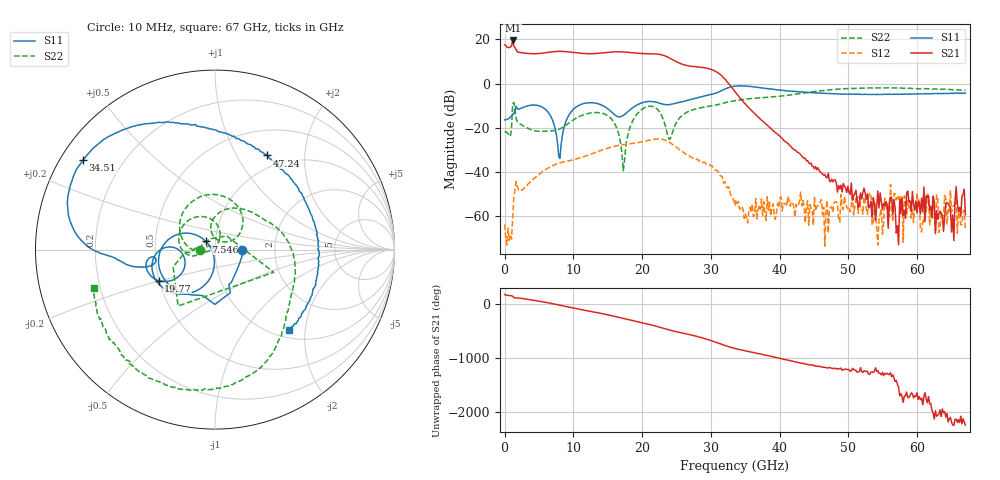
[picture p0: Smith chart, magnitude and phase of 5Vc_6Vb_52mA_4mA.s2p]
! MARKI MICROWAVE INC.
! Date:  05/05/2020
! Model Number:  APM-7099CH
! Description:  2-port Small Signal S-parameter data for APM-7099CH
! Frequency Range:  10 MHz to 67 GHz
! Port Configuration:  PORT 1: Input
!  PORT 2: Output
! Bias Condition: Vc = +5V, Vb = +6V
! APM-7099CH s2p files are only valid for small signal conditions (below -5 dBm input power)
!S2P File: Measurements: Mag<S11> Ang<S11>, Mag<S21> Ang<S21>, Mag<S12> Ang<S12>, Mag<S22> Ang<S22>!row 1
# Hz S  dB  R 50
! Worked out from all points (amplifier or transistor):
!   401 points, 10 MHz to 67 GHz, reference 50 ohm
!   highest |S21| = 19.6 dB at 1.182 GHz (marker M1)
!   |S21| within 3 dB of that: start of sweep to 376.6 MHz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
!   unconditionally stable (mu >= 1): start of sweep to end of sweep
!   at 11.06 GHz: K = 4.23, MAG = 14.4 dB, |S12| = -33.5 dB
!   at 33.51 GHz: K = 84.54, MAG = 3.5 dB, |S12| = -55.2 dB
!   at 67 GHz: K = 305005.63, MAG = -54.2 dB, |S12| = -66.6 dB
!   S11 on the Smith chart (normalised r, x): 10 MHz: 1.36, -0.01; 7.546 GHz: 0.90, +0.08; 19.77 GHz: 0.50, -0.20; 34.51 GHz: 0.06, +0.31; 47.24 GHz: 0.82, +1.35; 67 GHz: 1.14, -1.65
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1e7  -16.43 -0.7  17.58 178.4  -63.65 -92.9  -21.81 -179.2
1.182325e9  -13.79 -63.6  19.55 146.2  -60.90 85.2  -9.10 -21.1
1.68475e9  -10.30 -90.0  15.47 113.4  -44.32 -79.5  -15.57 -175.4
4.866775e9  -9.87 -168.9  13.61 58.7  -41.47 -175.8  -21.55 177.6
7.546375e9  -23.33 138.0  14.58 -6.3  -36.36 117.5  -21.04 -169.8
9.3886e9  -14.06 -105.1  14.36 -56.5  -34.96 76.4  -17.69 -164.1
1.123082e10  -9.24 -137.2  13.71 -102.6  -33.32 41.8  -14.41 176.9
1.3408e10  -8.94 -168.0  13.68 -154.4  -30.90 -2.1  -13.06 140.5
1.508275e10  -11.56 177.0  14.19 161.7  -29.15 -40.4  -14.67 103.8
1.74274e10  -14.01 -149.0  14.31 92.6  -27.53 -100.5  -35.18 179.7
1.977205e10  -8.91 -151.1  13.67 23.7  -26.47 -160.2  -12.13 142.5
2.111185e10  -8.04 -163.9  13.54 -16.8  -25.57 162.4  -10.22 98.7
2.245165e10  -8.75 -173.1  13.29 -62.4  -24.99 117.2  -12.41 50.2
2.47963e10  -8.94 -166.1  10.24 -143.5  -28.35 35.1  -18.77 101.5
2.848075e10  -6.03 -170.4  7.43 107.0  -34.89 -48.0  -10.93 50.2
3.065792e10  -4.35 -177.1  5.61 18.2  -39.20 -113.5  -9.73 29.6
3.3505e10  -1.14 158.0  -3.63 -99.0  -55.25 138.4  -7.68 5.4
3.450985e10  -1.03 146.0  -7.49 -128.9  -55.45 82.1  -7.19 -3.4
4.472582e10  -4.08 75.5  -37.41 -40.8  -57.63 -95.5  -3.68 -60.2
4.723795e10  -4.44 61.0  -44.06 -89.4  -57.07 -60.3  -2.79 -74.3
5.594665e10  -4.79 10.4  -53.58 135.1  -60.19 -147.9  -1.93 -117.9
6.7e10  -4.28 -47.5  -59.22 -74.0  -66.58 120.2  -3.00 -162.5
